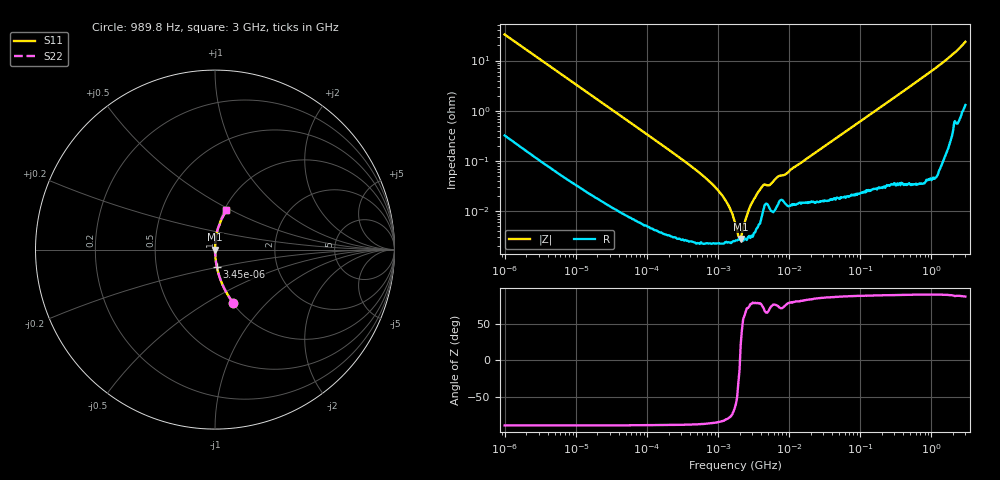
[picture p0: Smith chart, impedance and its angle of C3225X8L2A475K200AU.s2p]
! S-Parameter Data Generated by TDK Corporation
! Copyright(C) 2024 TDK Corporation.
! All Rights Reserved.
! TDK P/N: C3225X8L2A475K200AU (Multilayer Ceramic Chip Capacitor)
! Property: C=4.7uF
! Size(LxWxT): 3.2x2.5x2mm
! Model Type: s2p (Touchstone File Format Version 1.0)
! Frequency: DC=Yes Start=0.000989846MHz Stop=3000MHz 523points Log-sweep
! Model Generated on May 28, 2024
! Terms and conditions regarding TDK Simulation Models:
! 1)This simulation model is being provided solely for informational
!  purposes. Please refer to the specifications of the products in
!  terms of detailed characteristics of such products.
! 2)In no event shall TDK Corporation of any of its subsidiaries be
!  liable for any loss or damage arising, directly or indirectly,
!  from any information contained in this simulation model, including,
!  but not limited to loss or damages arising from any inaccuracies,
!  omissions or errors in connection with such information.
! 3)Any and all copyrights on this simulation model are owned by
!  TDK Corporation.  Duplication or redistribution of this simulation
!  model without prior written permission from TDK Corporation
!  is prohibited.
! 4)This simulation model is subject to any modification or change
!  without any prior notice.
! 5)Neither TDK Corporation nor any of its subsidiaries shall make any
!  warranty, express or implied, including but not limited to the
!  correctness, implied warranties of merchantability and fitness for
!  a particular purpose with respect to this simulation models.
! 6)The use of this simulation model shall be deemed to have consented
!  to the terms and conditions hereof.
! Port Assignments:
!  1 ---| |--- 2
! Applicable Conditions:
!  Temperature = 25 degC
!  DC Bias Voltage = 0 V
!  Small Signal Operation
# Hz S MA R 50
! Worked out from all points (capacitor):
!   522 points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, 989.8 Hz to 3 GHz, reference 50 ohm
!   read as one part in series: C = 4.85 uF near 1.07 kHz
!   lowest |Z| = 2.81 mohm at 2.074 MHz (marker M1)
!   series resonance near 2.027 MHz, so ESL is about 1.3 nH
!   S11 on the Smith chart (normalised r, x): 989.8 Hz: 1.01, -0.66; 3.45 kHz: 1.00, -0.19; 3 GHz: 1.03, +0.47
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989.846  0.313 -71.2  0.9467 18.2  0.9467 18.2  0.313 -71.2
1709.24  0.1886 -78.6  0.9802 10.9  0.9802 10.9  0.1886 -78.6
3450.01  0.09543 -84.0  0.9945 5.5  0.9945 5.5  0.09543 -84.0
12024.6  0.02777 -87.8  0.9993 1.6  0.9993 1.6  0.02777 -87.8
146075  0.002313 -88.9  1 0.1  1 0.1  0.002313 -88.9
669031  0.0004566 -87.1  1 0.0  1 0.0  0.0004566 -87.1
1068540  0.0002312 -84.4  1 0.0  1 0.0  0.0002312 -84.4
1518090  0.0001 -76.6  1 0.0  1 0.0  0.0001 -76.6
1774520  5.221e-05 -59.9  1 0.0  1 0.0  5.221e-05 -59.9
2074250  2.805e-05 21.7  1 -0.0  1 -0.0  2.805e-05 21.7
2424620  6.842e-05 65.5  1 -0.0  1 -0.0  6.842e-05 65.5
2621410  9.478e-05 71.2  1 -0.0  1 -0.0  9.478e-05 71.2
3444700  0.0002102 77.6  1 -0.0  1 -0.0  0.0002102 77.6
4186770  0.0003146 73.6  0.9999 -0.0  0.9999 -0.0  0.0003146 73.6
5291160  0.0003315 70.1  0.9999 -0.0  0.9999 -0.0  0.0003315 70.1
6952940  0.0004907 73.8  0.9999 -0.0  0.9999 -0.0  0.0004907 73.8
9136640  0.0005613 76.2  0.9999 -0.0  0.9999 -0.0  0.0005613 76.2
2.09559e7  0.001323 83.3  0.9998 -0.1  0.9998 -0.1  0.001323 83.3
2.50734e8  0.01536 87.9  0.9996 -0.9  0.9996 -0.9  0.01536 87.9
1.21884e9  0.0757 85.3  0.9966 -4.3  0.9966 -4.3  0.0757 85.3
2.17789e9  0.1456 79.3  0.9835 -8.4  0.9835 -8.4  0.1456 79.3
3e9  0.2275 73.7  0.9613 -13.1  0.9613 -13.1  0.2275 73.7
